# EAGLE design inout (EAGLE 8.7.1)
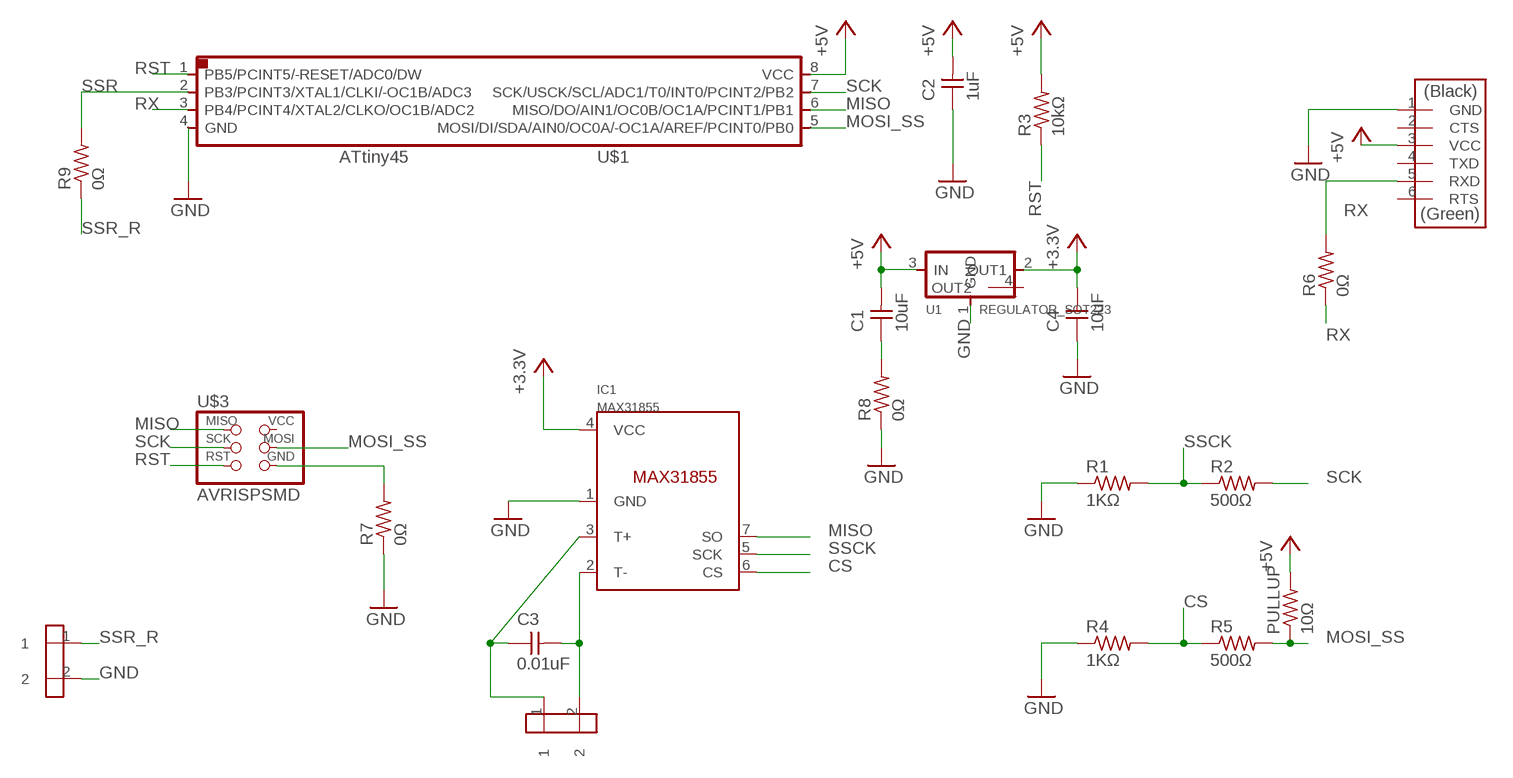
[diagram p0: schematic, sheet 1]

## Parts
C1  10uF  CAP-UNPOLARIZEDFAB  [C1206FAB]
C2  1uF  CAP-UNPOLARIZED  [C1206]
C3  0.01uF  CAP-UNPOLARIZEDFAB  [C1206FAB]
C4  10uF  CAP-UNPOLARIZEDFAB  [C1206FAB]
IC1  MAX31855  [SOIC8]
PULLUP  10Ω  RES-US1206FAB  [R1206FAB]
R1  1KΩ  RES-US1206FAB  [R1206FAB]
R2  500Ω  RES-US1206FAB  [R1206FAB]
R3  10kΩ  RES-US1206  [R1206]
R4  1KΩ  RES-US1206FAB  [R1206FAB]
R5  500Ω  RES-US1206FAB  [R1206FAB]
R6  0Ω  RES-US1206FAB  [R1206FAB]
R7  0Ω  RES-US1206FAB  [R1206FAB]
R8  0Ω  RES-US1206FAB  [R1206FAB]
R9  0Ω  RES-US1206FAB  [R1206FAB]
TML1  AKIZUKITNK_HOLE2PIN  [5.08PICH_HL]
TML2  AKIZUKITNK_HOLE2PIN  [5.08PICH_HL]
U1  REGULATOR_SOT223  [SOT223]
U$1  ATTINY45SI  [SOIC8]
U$2  FTDI-SMD-HEADER  [1X06SMD]
U$3  AVRISPSMD  [2X03SMD]

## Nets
3.3V: C4.2 IC1.4(VCC) U1.2(OUT1) ; supply symbol labelled +3.3V
+5V: C1.2 C2.2 PULLUP.2 R3.2 U1.3(IN) U$1.8(VCC) U$2.3(VCC)
CS: IC1.6(CS) R4.2 R5.1
GND: C1.1 C2.1 C4.1 IC1.1(GND) R1.1 R4.1 R7.1 R7.2 R8.1 R8.2 TML2.2 U1.1(GND) U$1.4(GND) U$2.1(GND) U$3.6(GND)
MISO: IC1.7(SO) U$1.6(MISO/DO/AIN1/OC0B/OC1A/PCINT1/PB1) U$3.1(MISO)
MOSI_SS: PULLUP.1 R5.2 U$1.5(MOSI/DI/SDA/AIN0/OC0A/-OC1A/AREF/PCINT0/PB0) U$3.4(MOSI)
N$2: C3.1 IC1.3(T+) TML1.1
N$3: C3.2 IC1.2(T-) TML1.2
RST: R3.1 U$1.1(PB5/PCINT5/-RESET/ADC0/DW) U$3.5(RST)
RX: R6.1 R6.2 U$1.3(PB4/PCINT4/XTAL2/CLKO/OC1B/ADC2) U$2.5(RXD)
SCK: R2.2 U$1.7(SCK/USCK/SCL/ADC1/T0/INT0/PCINT2/PB2) U$3.3(SCK)
SSCK: IC1.5(SCK) R1.2 R2.1
SSR: R9.2 U$1.2(PB3/PCINT3/XTAL1/CLKI/-OC1B/ADC3)
SSR_R: R9.1 TML2.1
Unconnected: U1.4(OUT2) U$2.2(CTS) U$2.4(TXD) U$2.6(RTS) U$3.2(VCC)

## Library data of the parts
C1-C4 = fab:CAP-UNPOLARIZED
IC1 = AlexW-Eagle-Libraries 2:MAX31855
PULLUP R1 R2 R4-R9 = fab:RES-US: Resistor (US Symbol)
R3 = HelloKamakura:RES-US: Resistor (US Symbol)
TML1 TML2 = doyo:AKIZUKI?TNK_HOLE2PIN
U1 = fab:REGULATOR_SOT223
U$1 = fab:ATTINY45
U$2 = fab:FTDI-SMD-HEADER
U$3 = HelloKamakura:AVRISP

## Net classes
0 default: width 0.406 mm

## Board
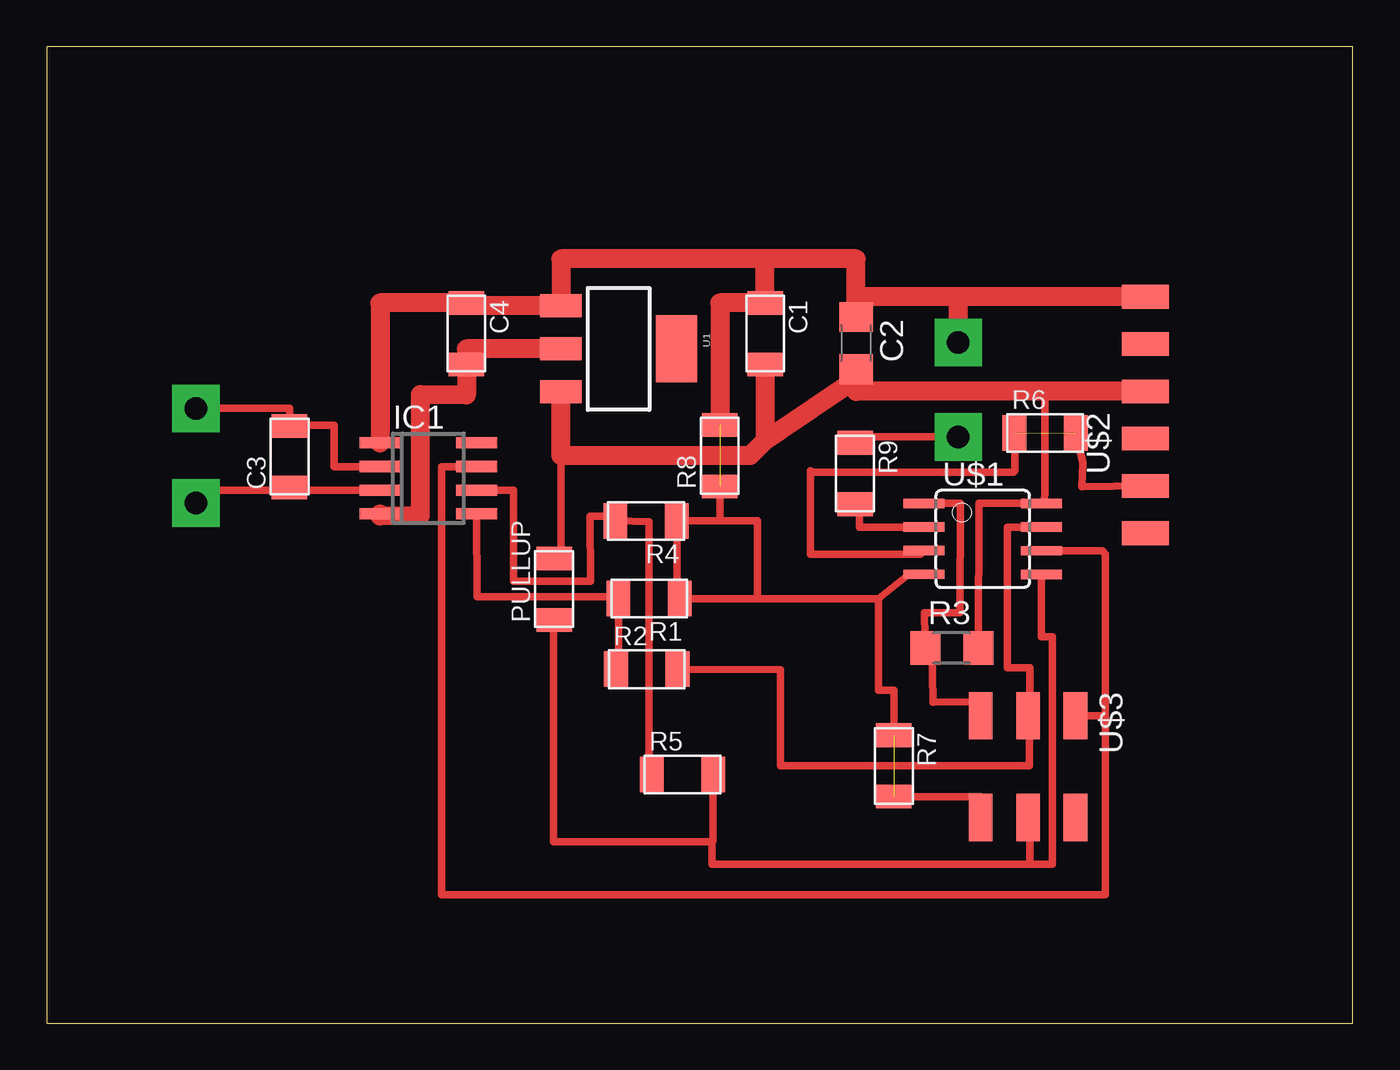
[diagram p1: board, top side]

Size 70.19 x 52.45 mm. Coordinates in mm from the lower left corner, seen from the top.
Outline: 0,0 70.19,0 70.19,52.45 0,52.45 0,0
Copper layers (1*16): Top 0.035mm / dielectric 1.5mm / Bottom 0.035mm
Design rules "default *": minimum track width 6mil, minimum drill 0.35mm, track to track 0.4mm, track to pad 0.4mm, pad to pad 0.4mm, via to via 0.4mm, smd to smd 0.4mm, copper to edge 40mil, drill to drill 6mil, minimum pad ring 10mil, minimum via ring 8mil, stop-mask expansion 4mil, vias tented up to drill 0mil, thermal gap 10mil

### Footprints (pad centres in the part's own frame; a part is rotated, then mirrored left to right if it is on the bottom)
C1206FAB = smd 1.27 x 1.905: 1 -1.651,0; 2 1.651,0
C1206 = smd 1.6 x 1.8: 1 -1.4,0; 2 1.4,0
SOIC8 = smd 0.6 x 2.2: 1 -1.905,-2.6; 2 -0.635,-2.6; 3 0.635,-2.6; 4 1.905,-2.6; 5 1.905,2.6; 6 0.635,2.6; 7 -0.635,2.6; 8 -1.905,2.6
R1206FAB = smd 1.27 x 1.905: 1 -1.651,0; 2 1.651,0
R1206 = smd 1.6 x 1.803: 1 -1.422,0; 2 1.422,0
5.08PICH_HL = drill 1.2 pad 2.54 square: 1 0,0; 2 -5.08,0
SOT223 = smd 1.219 x 2.235: 1 -2.311,-3.099; 2 0,-3.099; 3 2.311,-3.099 | smd 3.6 x 2.2: 4 0,3.099
SOIC8' = smd 0.5 x 2.2: 1 -1.905,-3.154; 2 -0.645,-3.154; 3 0.625,-3.154; 4 1.895,-3.154; 5 1.905,3.154; 6 0.635,3.154; 7 -0.635,3.154; 8 -1.905,3.154
1X06SMD = smd 2.54 x 1.27: 1 0,6.35; 2 0,3.81; 3 0,1.27; 4 0,-1.27; 5 0,-3.81; 6 0,-6.35
2X03SMD = smd 2.54 x 1.27: 1 -2.54,2.54; 2 2.92,2.54; 3 -2.54,0; 4 2.92,0; 5 -2.54,-2.54; 6 2.92,-2.54

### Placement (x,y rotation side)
C1  38.61,37.03 270 top
C2  43.48,36.53 270 top
C3  13.06,30.43 90 top
C4  22.56,37.03 270 top
IC1  20.51,29.26 270 top
PULLUP  27.27,23.31 90 top
R1  32.37,22.81 180 top
R2  32.25,19.01 0 top
R3  48.63,20.15 0 top
R4  32.21,26.97 180 top
R5  34.16,13.36 0 top
R6  53.64,31.7 0 top
R7  45.52,13.82 270 top
R8  36.17,30.48 90 top
R9  43.44,29.52 270 top
TML1  8.03,27.94 270 top
TML2  48.98,31.48 270 top
U1  30.73,36.22 270 top
U$1  ATTINY45SI  [SOIC8']  50.29,26.01 270 top
U$2  59.03,32.66 0 top
U$3  52.73,13.97 270 top

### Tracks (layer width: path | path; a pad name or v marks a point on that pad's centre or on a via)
3.3V
  Top 1.016: U1.2 22.55,36.22 C4.2 22.55,33.73 20.07,33.76 20.07,27.25 17.91,27.23 IC1.4
+5V
  Top 0.406: U$2.3 59.03,33.73 53.65,33.73 53.65,28.52 53.61,28.08 53.61,27.91 U$1.8 50.09,27.91 R3.2 | PULLUP.2 27.64,24.97 27.64,30.89
  Top 1.016: U$2.3 43.48,33.93 C2.2 43.66,34.72 38.61,31.29 | 38.61,31.29 37.8,30.48 27.64,30.48 27.64,30.89 U1.3 | C1.2 38.61,31.29
CS
  Top 0.406: R5.1 32.36,13.33 32.36,26.94 R4.2 30.56,27.23 29.21,27.23 29.21,23.72 25.09,23.72 25.08,28.63 IC1.6
GND  (2 unrouted)
  Top 0.406: 35.89,22.81 R1.1 | 44.7,22.81 38.2,22.81 | 38.2,22.81 R1.1 | U$1.4 46.33,24.11 44.7,22.81 | 38.2,22.81 38.2,26.98 36.17,26.98 | 36.17,26.98 R4.1 33.86,22.81 R1.1 | R7.2 50.19,12.17 U$3.6 | 44.7,22.81 44.7,17.88 45.52,17.88 R7.1 | 36.17,26.98 R8.1
  Top 1.016: U$2.1 48.77,39.01 | 48.77,39.01 43.48,39.01 | C2.1 43.48,39.01 | 43.48,39.01 43.48,41.05 38.61,41.05 | 38.61,41.05 27.64,41.05 U1.1 22.55,38.53 C4.1 17.91,38.68 IC1.1 | 38.61,41.05 C1.1 36.17,38.68 R8.2 | TML2.2 48.98,38.8 48.77,39.01
MISO
  Top 0.406: U$1.6 56.72,25.38 56.9,25.2 56.9,16.26 | 56.9,16.26 56.64,16.51 U$3.1 | 56.9,16.26 56.9,6.91 21.23,6.91 21.23,29.9 IC1.7
MOSI_SS
  Top 0.406: R5.2 35.81,9.8 | 35.81,9.8 35.76,9.75 27.23,9.75 27.23,21.62 PULLUP.1 | 35.81,9.8 35.76,9.8 35.76,8.53 52.83,8.53 | U$3.4 52.83,11.05 52.83,8.53 | U$1.5 53.45,20.77 54.02,20.77 54.02,8.53 52.83,8.53
N$2
  Top 0.406: IC1.3 13.87,28.63 | 13.87,28.63 C3.1 | TML1.1 8.84,28.63 13.87,28.63
N$3
  Top 0.406: IC1.2 15.44,29.9 15.44,32.11 13.06,32.11 C3.2 13.06,33.02 TML1.2
RST
  Top 0.406: 47.56,20.33 R3.1 47.2,20.73 47.17,22.03 49.06,22.03 49.09,27.91 U$1.1 | 47.56,20.33 47.61,17.24 50.19,17.27 U$3.5 | 47.14,20.74 47.56,20.33
RX  (1 unrouted)
  Top 0.406: 41.05,29.67 41.05,29.59 | 41.05,29.59 41.05,25.2 46.95,25.2 U$1.3 | R6.2 55.68,30.1 55.61,28.82 U$2.5 | R6.1 52.02,31.67 52.02,29.67 51.94,29.59 41.05,29.59
SCK
  Top 0.406: R2.2 39.42,18.99 39.42,13.82 52.79,13.82 52.79,16.26 | 52.79,16.26 52.79,16.51 U$3.3 | U$1.7 51.61,26.64 51.61,19.1 52.83,19.1 52.83,16.26 52.79,16.26
SSCK
  Top 0.406: IC1.5 23.14,22.9 30.75,22.9 R1.2 30.72,19.01 R2.1
SSR
  Top 0.406: R9.2 43.66,27.64 43.66,26.63 47.11,26.63 U$1.2
SSR_R
  Top 0.406: R9.1 43.74,31.48 TML2.1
